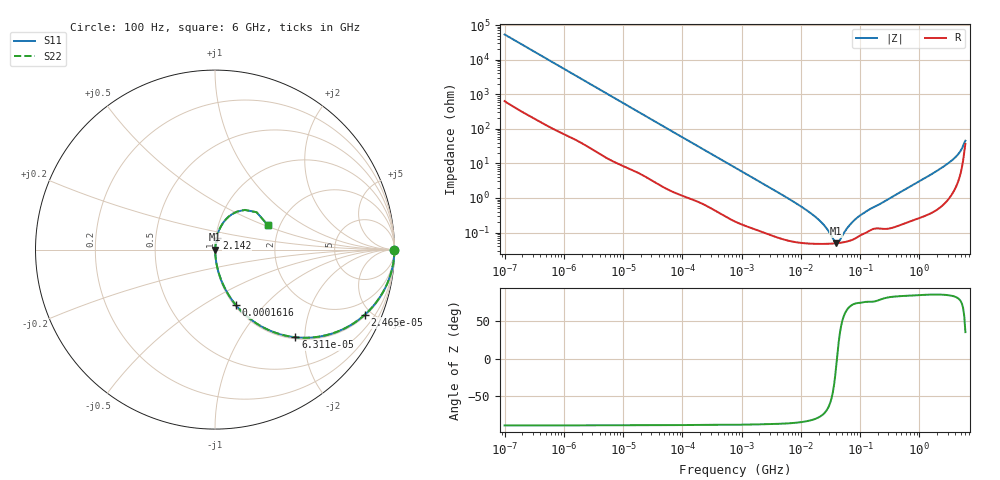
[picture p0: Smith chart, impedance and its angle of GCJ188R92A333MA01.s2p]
!Murata Part Number: GCJ188R92A333MA01
!These Parameters are Measured in Series Mode Connection
!Data Generated on Mar 13, 2026
!  o--ll--o
!Port1  Port2
!  o------o
!Operation Temp=25[degC], DC Bias Voltage=0[V]
!Freq. Start=100[Hz] Stop=6[GHz] 401[Steps]
# Hz S RI R 50
!Freq.(Hz) S11(Real) S11(Imag) S21(Real) S21(Imag) S12(Real) S12(Imag) S22(Real) S22(Imag)
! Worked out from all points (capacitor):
!   401 points, 100 Hz to 6 GHz, reference 50 ohm
!   read as one part in series: C = 29.6 nF near 109 Hz
!   lowest |Z| = 49.5 mohm at 39.84 MHz (marker M1)
!   series resonance near 40.76 MHz, so ESL is about 520 pH
!   S11 on the Smith chart (normalised r, x): 100 Hz: open; 24.65 kHz: 1.08, -4.56; 63.12 kHz: 1.03, -1.80; 161.6 kHz: 1.02, -0.71; 2.142 GHz: 1.01, +0.13; 6 GHz: 1.74, +0.53
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100  1 -0.00186  2.55e-05 0.00186  2.55e-05 0.00186  1 -0.00186
2008  0.9982 -0.0365  0.00185 0.0365  0.00185 0.0365  0.9982 -0.0365
7695  0.9793 -0.1355  0.0207 0.1355  0.0207 0.1355  0.9793 -0.1355
24648  0.8344 -0.3631  0.1656 0.3631  0.1656 0.3631  0.8344 -0.3631
40335  0.6599 -0.4652  0.3401 0.4652  0.3401 0.4652  0.6599 -0.4652
63115  0.4478 -0.4884  0.5522 0.4884  0.5522 0.4884  0.4478 -0.4884
103284  0.238 -0.4157  0.762 0.4157  0.762 0.4157  0.238 -0.4157
161617  0.1177 -0.3105  0.8823 0.3105  0.8823 0.3105  0.1177 -0.3105
345986  0.0316 -0.1621  0.9684 0.1621  0.9684 0.1621  0.0316 -0.1621
774597  0.00778 -0.0752  0.9922 0.0752  0.9922 0.0752  0.00778 -0.0752
6075234  0.00068 -0.00976  0.9993 0.00976  0.9993 0.00976  0.00068 -0.00976
1.555665e7  0.000485 -0.00334  0.9995 0.00334  0.9995 0.00334  0.000485 -0.00334
2.434276e7  0.000472 -0.00161  0.9995 0.00161  0.9995 0.00161  0.000472 -0.00161
3.983537e7  0.00049 -6.82e-05  0.9995 6.82e-05  0.9995 6.82e-05  0.00049 -6.82e-05
4.35672e7  0.000499 0.0002  0.9995 -0.0002  0.9995 -0.0002  0.000499 0.0002
6.233367e7  0.00056 0.00131  0.9994 -0.00131  0.9994 -0.00131  0.00056 0.00131
8.918374e7  0.000734 0.00258  0.9993 -0.00258  0.9993 -0.00258  0.000734 0.00258
3.124326e8  0.0014 0.00954  0.9986 -0.00954  0.9986 -0.00954  0.0014 0.00954
2.142435e9  0.00924 0.0651  0.9908 -0.0651  0.9908 -0.0651  0.00924 0.0651
4.385646e9  0.0516 0.1579  0.9484 -0.1579  0.9484 -0.1579  0.0516 0.1579
5.245841e9  0.1225 0.2115  0.8775 -0.2115  0.8775 -0.2115  0.1225 0.2115
6e9  0.2954 0.1352  0.7046 -0.1352  0.7046 -0.1352  0.2954 0.1352
